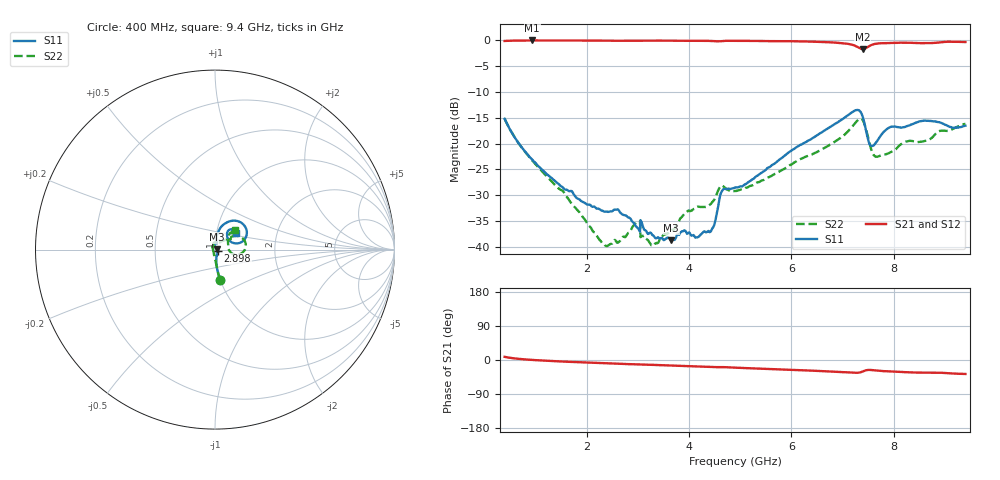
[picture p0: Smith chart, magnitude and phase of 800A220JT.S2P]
!  American Technical Ceramics  Date:  12/17/08
!  One Norden Lane
!  Huntington Station,  NY.  11746-2102
!  Tel:  (631) 622-4700  Fax:  (631) 622-4748
!  Part Number  800A220JT
!  Description: Broardband capacitor  Mounting Orientation: Vertical
!  Application:
# GHZ S DB R 50
! Freq  |S11|  S11 Ph  |S21|  S21 Ph  |S12|  S12 Ph  |S22|  S22 Ph
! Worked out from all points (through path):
!   801 points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, 400 MHz to 9.4 GHz, reference 50 ohm
!   highest |S21| = -0.08 dB at 940 MHz (marker M1); lowest = -1.8 dB at 7.398 GHz (marker M2)
!   group delay of S21, straight-line fit = 12.2 ps
!   lowest |S11| = -38.7 dB at 3.651 GHz (marker M3), VSWR 1.02, Z = 51.2 + j0.107 ohm
!   |S11| at or under -10 dB: start of sweep to end of sweep
!   |S22| runs from -39.8 to -15.2 dB; largest |S21 - S12| = 0.008
!   S11 on the Smith chart (normalised r, x): 400 MHz: 1.00, -0.35; 2.898 GHz: 1.03, -0.01; 9.4 GHz: 1.24, +0.23
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0.4  -15.21 -80.6  -0.18 8.4  -0.14 8.3  -15.19 -79.9
0.94  -23.11 -84.1  -0.08 0.2  -0.05 0.1  -23.29 -87.0
1.908  -31.18 -64.1  -0.09 -6.3  -0.06 -6.4  -33.90 -110.3
2.391  -33.12 -39.8  -0.12 -8.9  -0.09 -9.0  -39.82 -157.0
2.594  -32.74 -32.8  -0.14 -9.8  -0.11 -9.9  -39.15 163.6
2.898  -35.09 -23.5  -0.15 -11.2  -0.12 -11.3  -36.08 130.9
2.999  -36.32 -16.4  -0.16 -11.6  -0.13 -11.8  -35.07 120.3
3.1  -35.98 -45.8  -0.15 -11.9  -0.12 -12.1  -37.80 135.5
3.258  -37.27 -28.4  -0.13 -12.7  -0.10 -12.8  -39.53 130.2
3.404  -38.16 -15.6  -0.11 -13.4  -0.09 -13.6  -39.11 143.7
3.651  -38.71 5.2  -0.13 -14.7  -0.10 -14.9  -36.87 140.1
3.955  -37.27 22.1  -0.15 -16.1  -0.12 -16.3  -33.23 132.0
4.428  -36.96 73.1  -0.18 -18.4  -0.16 -18.6  -31.67 110.9
4.653  -29.05 85.3  -0.20 -18.7  -0.18 -18.9  -28.15 89.4
4.9  -28.51 72.3  -0.14 -20.2  -0.13 -20.4  -29.15 73.1
6.408  -18.99 78.0  -0.32 -28.1  -0.32 -28.4  -22.07 43.0
7.24  -13.63 47.2  -1.08 -33.8  -1.09 -34.1  -16.13 27.4
7.398  -14.91 20.3  -1.76 -30.1  -1.77 -30.4  -15.53 0.6
7.566  -20.45 35.0  -0.95 -26.4  -0.97 -26.8  -21.30 -8.6
7.904  -16.96 52.5  -0.58 -30.0  -0.60 -30.4  -21.86 26.5
8.613  -15.59 41.8  -0.61 -33.4  -0.64 -33.8  -19.49 40.6
9.4  -16.55 37.5  -0.38 -36.9  -0.42 -37.3  -16.20 43.6
